{attribute 'Tc2GvlVarNames'}
(* Generated automatically by TwinCAT - (read only) *)
VAR_CONFIG
	MAIN.master.PlcToNc AT %QB0 : PLCTONC_AXIS_REF;
	MAIN.master.NcToPlc AT %IB1 : NCTOPLC_AXIS_REF;
	MAIN.slave.PlcToNc AT %QB128 : PLCTONC_AXIS_REF;
	MAIN.slave.NcToPlc AT %IB129 : NCTOPLC_AXIS_REF;
	MAIN.bEL1259_input AT %IX0.0 : BOOL;
END_VAR
